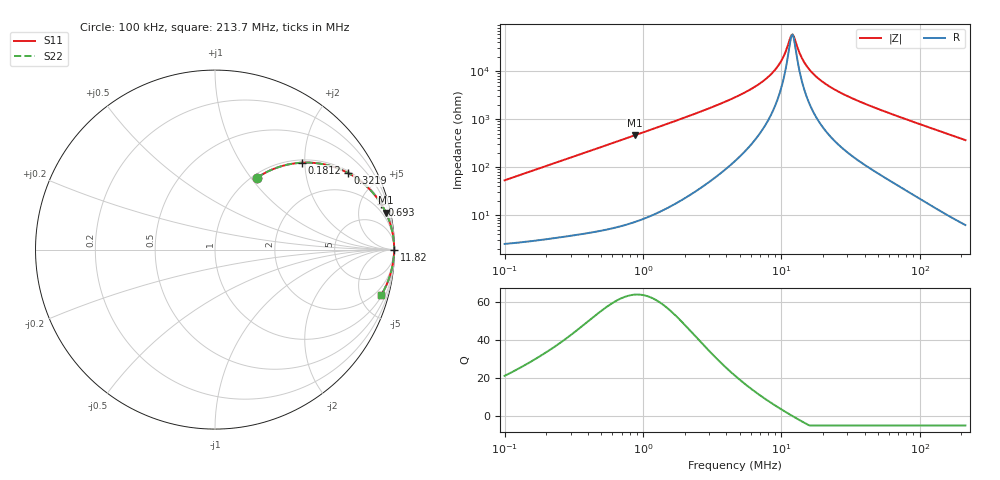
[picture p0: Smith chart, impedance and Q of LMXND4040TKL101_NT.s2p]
! LMXND4040TKL101_NT  S-PARAMETER MODEL  ( Standard Model )
! Model Generated by TAIYO YUDEN Corporation (https://www.yuden.co.jp/en/)
! Version 1.0
! TAIYO YUDEN Control No. 20250409
! Copyright(c) 2025 TAIYO YUDEN CO.,LTD. All Rights Reserved.
! Product Description (link to TY-COMPAS)
! https://ds.yuden.co.jp/TYCOMPAS/or/detail?pn=LMXND4040TKL101MNT&u=M
! Products Name : Inductors
! Characteristics :
!  Inductance : 100 [uH] , SRF(min) : 6.5 [MHz] , DC Resistance(max) : 1.74 [Ohm]
!  Rated Current : Saturation  420 [mA] , Temp Rise  470 [mA] (40 [degC])
!  Case Size : 4.0 x 4.0 / 0.157 x 0.157 [mm/inch] , Thickness : 1.8 / 0.071 [mm/inch]
!  (Conditions: Temperature = 25 [degC] , DC Bias Current = 0 [A])
! External Node Assignments :
!  1  o---GGG---o  2
! GND o---------o GND
! Frequency Range : 0.1MHz  -  213.673535MHz  [ 402 STEP ]
# MHz S RI R 50
! Freq[MHz].  S11 Real  S11 Imag  S21 Real  S21 Imag  S12 Real  S12 Imag  S22 Real  S22 Imag
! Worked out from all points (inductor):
!   401 points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, 100 kHz to 213.7 MHz, reference 50 ohm
!   read as one part in series: L = 85 uH near 103.9 kHz
!   highest Q = 63.9 at 872.3 kHz (marker M1), where L = 84.5 uH
!   self-resonance near 11.82 MHz
!   S11 on the Smith chart (normalised r, x): 100 kHz: 1.05, +1.07; 181.2 kHz: 1.06, +1.93; 321.9 kHz: 1.08, +3.42; 693 kHz: 1.12, +7.35; 11.82 MHz: open; 213.7 MHz: 1.13, -7.36
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0.1  0.2339 0.4003  0.7661 -0.4003  0.7661 -0.4003  0.2339 0.4003
0.181157  0.4832 0.4841  0.5168 -0.4841  0.5168 -0.4841  0.4832 0.4841
0.321949  0.7402 0.4274  0.2598 -0.4274  0.2598 -0.4274  0.7402 0.4274
0.361188  0.781 0.4031  0.219 -0.4031  0.219 -0.4031  0.781 0.4031
0.693046  0.9275 0.2513  0.0725 -0.2513  0.0725 -0.2513  0.9275 0.2513
0.872277  0.9525 0.205  0.0475 -0.205  0.0475 -0.205  0.9525 0.205
1.304567  0.9776 0.1399  0.0224 -0.1399  0.0224 -0.1399  0.9776 0.1399
2.808288  0.9942 0.0633  0.00577 -0.0633  0.00577 -0.0633  0.9942 0.0633
4.71194  0.9972 0.0339  0.00279 -0.0339  0.00279 -0.0339  0.9972 0.0339
6.78208  0.998 0.0189  0.00199 -0.0189  0.00199 -0.0189  0.998 0.0189
8.701213  0.9982 0.0103  0.00176 -0.0103  0.00176 -0.0103  0.9982 0.0103
10.1432  0.9983 0.00531  0.0017 -0.00531  0.0017 -0.00531  0.9983 0.00531
11.82415  0.9983 0.000465  0.0017 -0.000465  0.0017 -0.000465  0.9983 0.000465
12.28623  0.9983 -0.00074  0.00171 0.00074  0.00171 0.00074  0.9983 -0.00074
13.52199  0.9982 -0.00376  0.00175 0.00376  0.00175 0.00376  0.9982 -0.00376
14.32233  0.9982 -0.00558  0.00179 0.00558  0.00179 0.00558  0.9982 -0.00558
16.69585  0.9981 -0.0105  0.00193 0.0105  0.00193 0.0105  0.9981 -0.0105
20.22332  0.9978 -0.0171  0.0022 0.0171  0.0022 0.0171  0.9978 -0.0171
26.44805  0.9972 -0.0273  0.00285 0.0273  0.00285 0.0273  0.9972 -0.0273
60.30341  0.9915 -0.0738  0.00846 0.0738  0.00846 0.0738  0.9915 -0.0738
115.7099  0.9756 -0.1423  0.0244 0.1423  0.0244 0.1423  0.9756 -0.1423
213.6735  0.9276 -0.2508  0.0724 0.2508  0.0724 0.2508  0.9276 -0.2508
